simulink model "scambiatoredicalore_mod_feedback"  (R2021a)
settings: Solver=FixedStepAuto  StartTime=0.0  StopTime=18000  FixedStep=Tsim  MaxStep=1  RelTol=1e-3
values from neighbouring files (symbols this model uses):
  ca = 4178    [scambiatoredicalore_dati.m]    (also in scambiatoremodelloTD.m)
  cb = 2131    [scambiatoredicalore_dati.m]    (also in scambiatoremodelloTD.m)
  Ki = 2287    [scambiatoredicalore_dati.m]    (also in scambiatoremodelloTD.m)
  ma = rhoa*pi*Di^2/4*L    (= 38.4179965995)    [scambiatoredicalore_dati.m]    (also in scambiatoremodelloTD.m)
  mb = rhob*pi*(Dan^2-De^2)/4*L    (= 72.0857488137)    [scambiatoredicalore_dati.m]    (also in scambiatoremodelloTD.m)
  Rba = Ri+Re+Rparete    [scambiatoredicalore_dati.m]    (also in scambiatoremodelloTD.m)
  Ta0 = 35    [scambiatoremodelloTD.m]
  Tain = 30    [scambiatoredicalore_dati.m]    (also in scambiatoremodelloTD.m)
  Tb0 = 55    [scambiatoremodelloTD.m]
  Tbin = 100    [scambiatoredicalore_dati.m]    (also in scambiatoremodelloTD.m)
  wa = 0.2    [scambiatoredicalore_dati.m]    (also in scambiatoremodelloTD.m)
  wb = 0.1    [scambiatoredicalore_dati.m]    (also in scambiatoremodelloTD.m)
undefined symbols (not defined in the file or in its folder): Kp, Tbin2
libraries: pid_lib x1

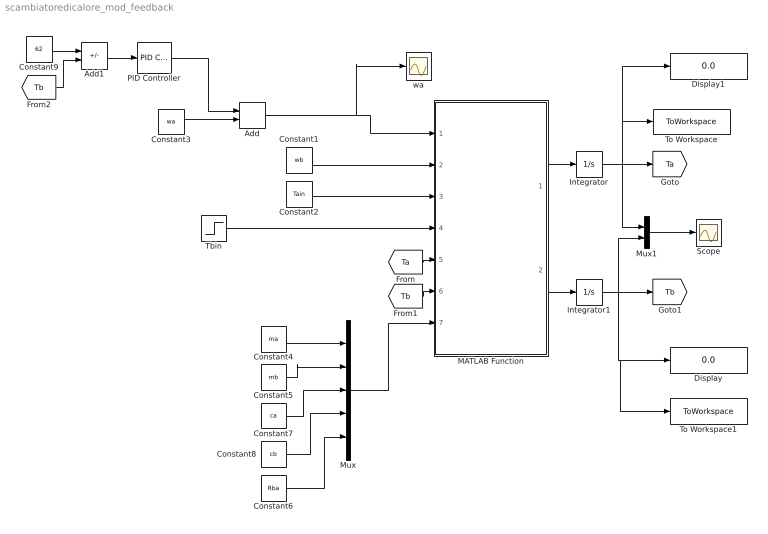
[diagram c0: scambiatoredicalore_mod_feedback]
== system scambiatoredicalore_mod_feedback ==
  Add : Sum
  Add1 : Sum  Inputs=-+
  Constant1 : Constant  Value=wb
  Constant2 : Constant  Value=Tain
  Constant3 : Constant  Value=wa
  Constant4 : Constant  Value=ma
  Constant5 : Constant  Value=mb
  Constant6 : Constant  Value=Rba
  Constant7 : Constant  Value=ca
  Constant8 : Constant  Value=cb
  Constant9 : Constant  Value=62
  Display : Display
  Display1 : Display
  Integrator : Integrator  InitialCondition=Ta0
  Integrator1 : Integrator  InitialCondition=Tb0
  MATLAB Function : MATLAB Function  TreatAsAtomicUnit=on
  Mux : Mux  Inputs=5
  Mux1 : Mux  Inputs=2
  PID Controller : pid_lib/PID Controller  Controller=PID  Form=Parallel  TimeDomain=Continuous-time  UseExternalTs=off  SampleTime=-1  IntegratorMethod=Forward Euler  FilterMethod=Forward Euler  ControllerParametersSource=internal  P=Kp  I=Ki  D=0  UseFilter=on  N=100  TunerSelectOption=Transfer Function Based (PID Tuner App)  InitialConditionSource=internal  InitialConditionForIntegrator=0  InitialConditionForFilter=0  DifferentiatorICPrevScaledInput=0  ExternalReset=none  TrackingMode=off  Kt=1  LimitOutput=off  SatLimitsSource=internal  UpperSaturationLimit=inf  LowerSaturationLimit=-inf  LinearizeAsGain=on  AntiWindupMode=none  Kb=1  POutMin=[]  POutMax=[]  IOutMin=[]  IOutMax=[]  DOutMin=[]  DOutMax=[]  NOutMin=[]  NOutMax=[]  SumOutMin=[]  SumOutMax=[]  SaturationOutMin=[]  SaturationOutMax=[]  PParamMin=[]  PParamMax=[]  IParamMin=[]  IParamMax=[]  DParamMin=[]  DParamMax=[]  NParamMin=[]  NParamMax=[]  KbParamMin=[]  KbParamMax=[]  KtParamMin=[]  KtParamMax=[]  KbOutMin=[]  KbOutMax=[]  KtOutMin=[]  KtOutMax=[]  IntegratorOutMin=[]  IntegratorOutMax=[]  FilterOutMin=[]  FilterOutMax=[]  SumI1OutMin=[]  SumI1OutMax=[]  SumI2OutMin=[]  SumI2OutMax=[]  SumI3OutMin=[]  SumI3OutMax=[]  SumI4OutMin=[]  SumI4OutMax=[]  SumDOutMin=[]  SumDOutMax=[]  DifferentiatorOutMin=[]  DifferentiatorOutMax=[]  FilterDiffOutCoefMin=[]  FilterDiffOutCoefMax=[]  ReciprocalOutMin=[]  ReciprocalOutMax=[]  SumDenOutMin=[]  SumDenOutMax=[]  SumNumOutMin=[]  SumNumOutMax=[]  DivideOutMin=[]  DivideOutMax=[]  UdiffTsProdOutMin=[]  UdiffTsProdOutMax=[]  NTsProdOutMin=[]  NTsProdOutMax=[]  UintegralTsProdOutMin=[]  UintegralTsProdOutMax=[]  UngainTsProdOutMin=[]  UngainTsProdOutMax=[]  IntegratorContinuousStateAttributes=''  IntegratorStateMustResolveToSignalObject=off  IntegratorRTWStateStorageClass=Auto  FilterContinuousStateAttributes=''  FilterStateMustResolveToSignalObject=off  FilterRTWStateStorageClass=Auto  ParallelPVariant=InternalParameters  IdealPVariant=Disabled  IVariant=InternalParameters  DVariant=InternalParameters  IntegratorVariant=Continuous  SatVariant=Disabled  AWVariant=Passthrough  PCopyVariant=Disabled  TRVariant=Disabled  FdbkBlocksVariant=Forward  IdealPFdbkVariant=Disabled  SatFdbkVariant=Disabled  DerivativeFilterVariant=ContFilter  NVariant=InternalParameters  NCopyVariant=Disabled  FilterICVariant=InternalICsFilter  IntegratorICVariant=InternalICs  ExternalResetVariant=Disabled  TRSumVariant=Passthrough  SumFdbkVariant=Disabled  SumVariant=Sum_PID  TsampFilterVariant=InternalTs  TsampNgainVariant=Passthrough  TsampIntegralVariant=Passthrough  ExternalSaturationOutDataTypeStr=Inherit: Same as second input
  Scope : Scope
  Tbin : Step  Time=10000  Before=Tbin  After=Tbin2  SampleTime=0
  To Workspace : ToWorkspace  VariableName=TaFb  SaveFormat=Timeseries  SampleTime=-1
  To Workspace1 : ToWorkspace  VariableName=TbFb  SaveFormat=Timeseries  SampleTime=-1
  wa : Scope
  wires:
  MATLAB Function/1(Tadot) -> Integrator/1
  MATLAB Function/2(Tbdot) -> Integrator1/1
  Integrator/1 -> [Ta], Display1/1, To Workspace/1, Mux1/1
  Integrator1/1 -> To Workspace1/1, Display/1, Mux1/2, [Tb]
  [Ta] -> MATLAB Function/5(Ta)
  [Tb] -> MATLAB Function/6(Tb)
  Add/1 -> wa/1, MATLAB Function/1(wa)
  Constant1/1 -> MATLAB Function/2(wb)
  Constant2/1 -> MATLAB Function/3(Tain)
  Tbin/1 -> MATLAB Function/4(Tbin)
  Constant4/1 -> Mux/1
  Constant5/1 -> Mux/2
  Mux/1 -> MATLAB Function/7(par)
  Constant7/1 -> Mux/3
  Constant8/1 -> Mux/4
  Constant6/1 -> Mux/5
  Mux1/1 -> Scope/1
  Constant3/1 -> Add/2
  [Tb] -> Add1/2
  Constant9/1 -> Add1/1
  Add1/1 -> PID Controller/1
  PID Controller/1 -> Add/1

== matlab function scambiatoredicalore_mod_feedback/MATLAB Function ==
function [Tadot,Tbdot] = fcn(wa,wb,Tain,Tbin,Ta,Tb,par)

ma=par(1);
mb=par(2);
ca=par(3);
cb=par(4);
Rba=par(5);

DT1=Tbin-Ta;
DT2=Tb-Tain;

Tadot =  1/ma*wa*(Tain-Ta)+1/(Rba*ma*ca)*(DT1-DT2)/log(DT1/DT2);
Tbdot =  1/mb*wb*(Tbin-Tb)-1/(Rba*mb*cb)*(DT1-DT2)/log(DT1/DT2);
